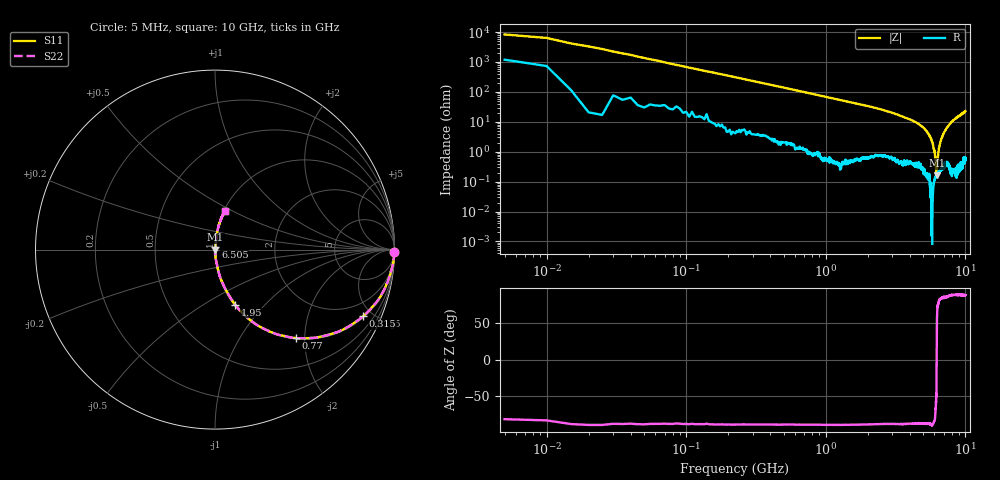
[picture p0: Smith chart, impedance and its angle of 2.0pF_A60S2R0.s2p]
! Amotech Co.,Ltd.
! http://www.amotech.co.kr/
! Part Number: A60S2R0
! These Parameters are Measured in Series Mode Connection
! Operation Temp=25[degC], DC Bias Voltage=0[V]
! Freq. Start=5[MHz] Stop=10[GHz], 2000[Steps]
! Date: Monday, July 13, 2020, 01:51:18
# GHZ S RI R 50.000000
!Freq.(Hz) S11(Real) S11(Imag) S21(Real) S21(Imag) S12(Real) S12(Imag) S22(Real) S22(Imag)
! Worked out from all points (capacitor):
!   2000 points, 5 MHz to 10 GHz, reference 50 ohm
!   read as one part in series: C = 2.33 pF near 55 MHz
!   lowest |Z| = 164 mohm at 6.225 GHz (marker M1)
!   series resonance near 6.224 GHz, so ESL is about 280 pH
!   S11 on the Smith chart (normalised r, x): 5 MHz: open; 315 MHz: 1.07, -4.40; 770 MHz: 1.02, -1.80; 1.95 GHz: 1.01, -0.69; 6.505 GHz: 1.00, +0.03; 10 GHz: 1.01, +0.46
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0.005  0.9981 -0.0118  0.00186 0.0118  0.00186 0.0118  0.9981 -0.0118
0.07  0.9859 -0.1006  0.0141 0.1006  0.0141 0.1006  0.9859 -0.1006
0.11  0.9694 -0.1555  0.0306 0.1555  0.0306 0.1555  0.9694 -0.1555
0.195  0.9242 -0.2582  0.0758 0.2582  0.0758 0.2582  0.9242 -0.2582
0.315  0.825 -0.3717  0.175 0.3717  0.175 0.3717  0.825 -0.3717
0.77  0.4493 -0.4924  0.5507 0.4924  0.5507 0.4924  0.4493 -0.4924
1.175  0.2566 -0.4335  0.7434 0.4335  0.7434 0.4335  0.2566 -0.4335
1.675  0.1455 -0.3457  0.8545 0.3457  0.8545 0.3457  0.1455 -0.3457
1.95  0.1117 -0.3064  0.8883 0.3064  0.8883 0.3064  0.1117 -0.3064
3.34  0.0308 -0.1603  0.9692 0.1603  0.9692 0.1603  0.0308 -0.1603
5.005  0.00601 -0.0628  0.994 0.0628  0.994 0.0628  0.00601 -0.0628
5.585  0.00169 -0.0324  0.9983 0.0324  0.9983 0.0324  0.00169 -0.0324
5.825  0.000631 -0.0197  0.9994 0.0197  0.9994 0.0197  0.000631 -0.0197
6.03  0.00129 -0.00985  0.9987 0.00985  0.9987 0.00985  0.00129 -0.00985
6.18  0.00155 -0.00214  0.9984 0.00214  0.9984 0.00214  0.00155 -0.00214
6.225  0.00164 8.96e-05  0.9984 -8.96e-05  0.9984 -8.96e-05  0.00164 8.96e-05
6.32  0.00177 0.00598  0.9982 -0.00598  0.9982 -0.00598  0.00177 0.00598
6.505  0.00237 0.0148  0.9976 -0.0148  0.9976 -0.0148  0.00237 0.0148
6.67  0.00308 0.023  0.9969 -0.023  0.9969 -0.023  0.00308 0.023
7.29  0.00699 0.0577  0.993 -0.0577  0.993 -0.0577  0.00699 0.0577
8.335  0.0163 0.1179  0.9837 -0.1179  0.9837 -0.1179  0.0163 0.1179
10  0.0546 0.2152  0.9454 -0.2152  0.9454 -0.2152  0.0546 0.2152
